(* Logix 5000 AddOnInstructionDefinition export SPEL_Jump; software revision 30.01 *)

ADD_ON_INSTRUCTION SPEL_ExecCmd   (* revision 1.0 *)
// Executes a command in the robot controller.  Normally this is called by higher level AOIs.
VAR_INPUT
   Start : BOOL; {required}
   MaxTime : DINT := 3000; {required}
END_VAR
VAR_OUTPUT
   InCycle : BOOL; {access Read Only, visible}
   Done : BOOL; {access Read Only, visible}
   Error : BOOL; {access Read Only, visible}
END_VAR
VAR_IN_OUT
   ExtInputs : AB:ETHERNET_MODULE_INT_128Bytes:I:0; {required}
        .DATA[0].0   // ExtCmdGet
        .DATA[0].1   // ExtRespSet
        .DATA[0].2   // ExtCmdResult
        .DATA[0].3   // ExtError
   ExtOutputs : AB:ETHERNET_MODULE_INT_128Bytes:O:0; {required}
        .DATA[0].0   // ExtCmdSet
        .DATA[0].1   // ExtRespGet
        .DATA[0].2   // ExtCmdReset
END_VAR
VAR_INPUT
   Cmd : INT; {required}
   CmdParam1 : INT; {required}
   CmdParam2 : INT; {required}
   CmdParam3 : INT; {required}
   CmdParam4 : INT; {required}
   CmdParam5 : INT; {required}
   CmdParam6 : INT; {required}
   CmdParam7 : INT; {required}
END_VAR
VAR_OUTPUT
   CmdEcho : INT; {access Read Only, visible}
   Resp1 : INT; {access Read Only, visible}
   Resp2 : INT; {access Read Only, visible}
   Resp3 : INT; {access Read Only, visible}
   Resp4 : INT; {access Read Only, visible}
   Resp5 : INT; {access Read Only, visible}
   Resp6 : INT; {access Read Only, visible}
   Resp7 : INT; {access Read Only, visible}
   ErrCode1 : INT; {access Read Only, visible}
   ErrCode2 : INT; {access Read Only, visible}
END_VAR
VAR
   ExtReset : BOOL; {access None}
   ExtError : BOOL; {access None}
   ExtCmdSet : BOOL; {access None}   // Cmd Ready
   ExtCmdGet : BOOL; {access None}   // Cmd Received
   CmdXferDone : BOOL; {access None}
   ExtRespSet : BOOL; {access None}   // Resp Ready
   RespXferDone : BOOL; {access None}
   ExtCmdResult : BOOL; {access None}   // Normal or Error?
   TmrCmdDataRdy : TIMER := (PRE := 5); {access None}
   OneShotDoneOff : BOOL; {access None}
   OneShotStart : BOOL; {access None}
   StartInit : BOOL; {access None}
   OneShotStartError : BOOL; {access None}
   TmrCycle : TIMER := (PRE := 5000); {access None}
   OneshotTmrPreset : BOOL; {access None}
   TmrCmdSet : TIMER := (PRE := 20); {access None}
   OnShotCmdDataXfer : BOOL; {access None}
   OneShotRespDataXfer : BOOL; {access None}
   OneShotDataRdy : BOOL; {access None}
   OtherCmdInCycle : BOOL; {access None}
   s : BOOL; {access None}
   OneShotUnsetCmdIncycle : BOOL; {access None}
   OneShotSetCmdIncycle : BOOL; {access None}
   OneShotSetOtherCmdInCycleError : BOOL; {access None}
   OneShotSetBit : BOOL; {access None}
   MaxTimeError : BOOL; {access None}
END_VAR

ROUTINE Logic   (* ladder *)
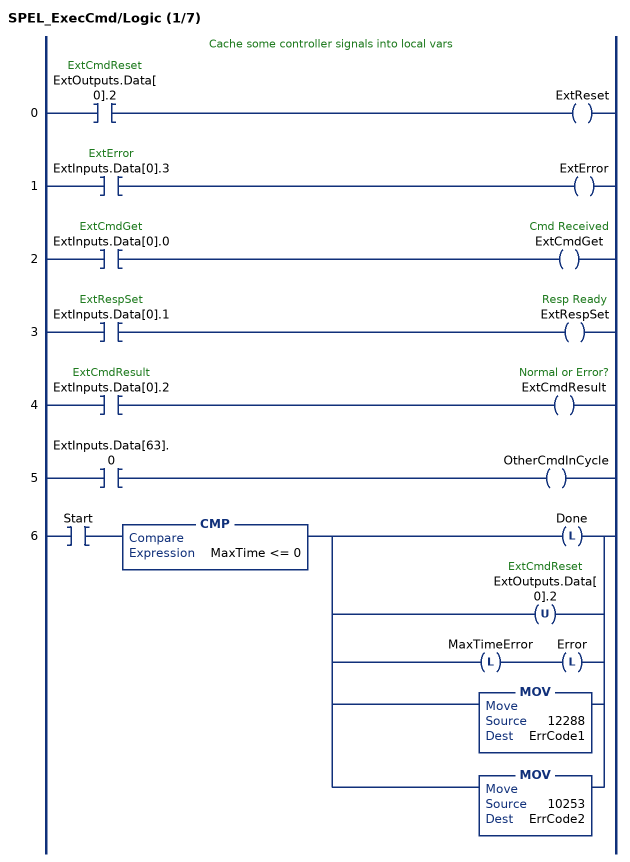
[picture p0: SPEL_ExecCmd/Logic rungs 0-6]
   // Cache some controller signals into local vars
   0: XIC(ExtOutputs.Data[0].2)OTE(ExtReset);
   1: XIC(ExtInputs.Data[0].3)OTE(ExtError);
   2: XIC(ExtInputs.Data[0].0)OTE(ExtCmdGet);
   3: XIC(ExtInputs.Data[0].1)OTE(ExtRespSet);
   4: XIC(ExtInputs.Data[0].2)OTE(ExtCmdResult);
   5: XIC(ExtInputs.Data[63].0)OTE(OtherCmdInCycle);
   6: XIC(Start)CMP(MaxTime <= 0)[OTL(Done) ,OTU(ExtOutputs.Data[0].2) ,OTL(MaxTimeError) OTL(Error) ,MOV(12288,ErrCode1) ,MOV(10253,ErrCode2) ];
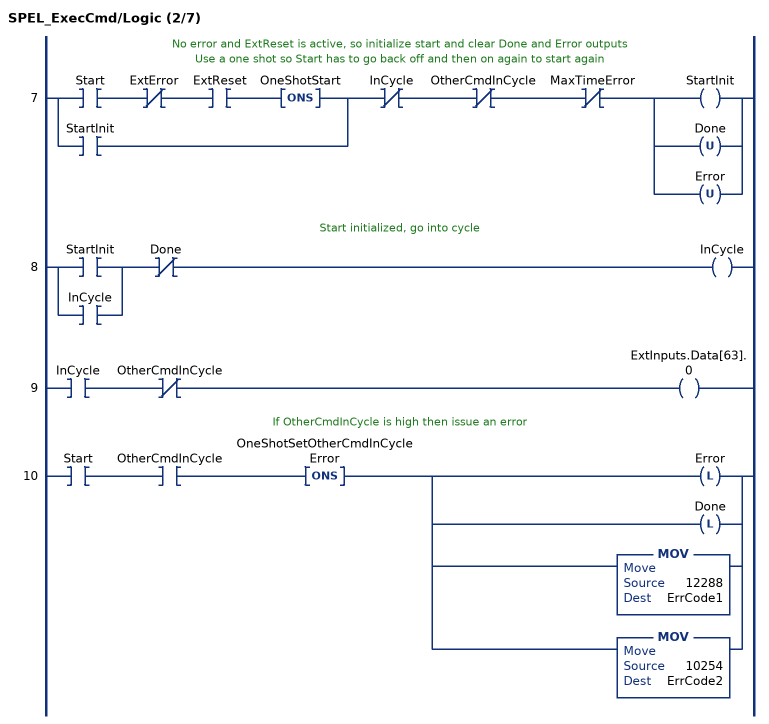
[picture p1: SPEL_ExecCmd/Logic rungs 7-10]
   // No error and ExtReset is active, so initialize start and clear Done and Error outputs
   // Use a one shot so Start has to go back off and then on again to start again
   7: [XIC(Start) XIO(ExtError) XIC(ExtReset) ONS(OneShotStart) ,XIC(StartInit) ]XIO(InCycle)XIO(OtherCmdInCycle)XIO(MaxTimeError)[OTE(StartInit) ,OTU(Done) ,OTU(Error) ];
   // Start initialized, go into cycle
   8: [XIC(StartInit) ,XIC(InCycle) ]XIO(Done)OTE(InCycle);
   9: XIC(InCycle)XIO(OtherCmdInCycle)OTE(ExtInputs.Data[63].0);
   // If OtherCmdInCycle is high then issue an error
   10: XIC(Start)XIC(OtherCmdInCycle)ONS(OneShotSetOtherCmdInCycleError)[OTL(Error) ,OTL(Done) ,MOV(12288,ErrCode1) ,MOV(10254,ErrCode2) ];
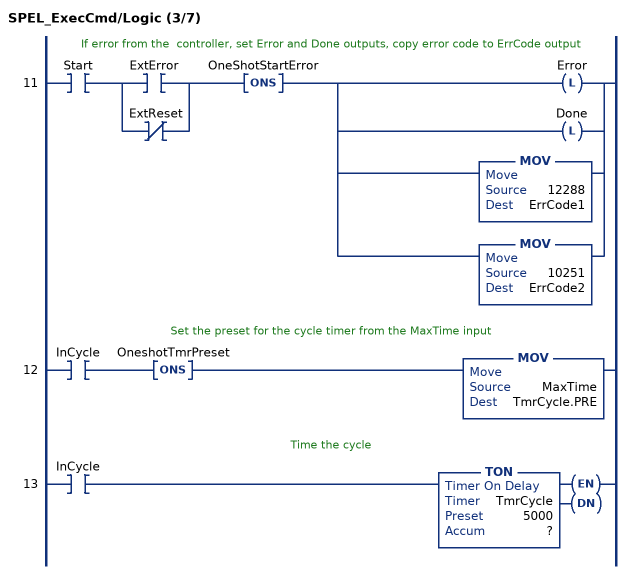
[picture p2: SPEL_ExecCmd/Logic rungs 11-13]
   // If error from the  controller, set Error and Done outputs, copy error code to ErrCode output
   11: XIC(Start)[XIC(ExtError) ,XIO(ExtReset) ]ONS(OneShotStartError)[OTL(Error) ,OTL(Done) ,MOV(12288,ErrCode1) ,MOV(10251,ErrCode2) ];
   // Set the preset for the cycle timer from the MaxTime input
   12: XIC(InCycle)ONS(OneshotTmrPreset)MOV(MaxTime,TmrCycle.PRE);
   // Time the cycle
   13: XIC(InCycle)TON(TmrCycle,?,?);
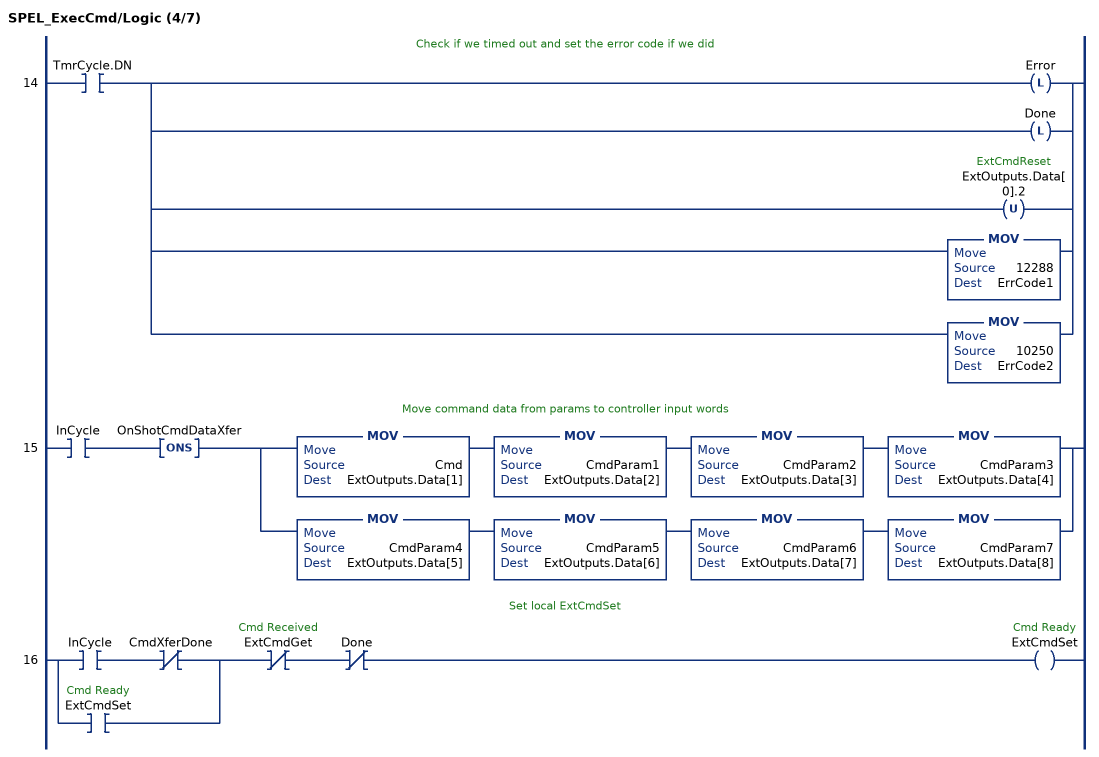
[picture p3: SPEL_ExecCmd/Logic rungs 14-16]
   // Check if we timed out and set the error code if we did
   14: XIC(TmrCycle.DN)[OTL(Error) ,OTL(Done) ,OTU(ExtOutputs.Data[0].2) ,MOV(12288,ErrCode1) ,MOV(10250,ErrCode2) ];
   // Move command data from params to controller input words
   15: XIC(InCycle)ONS(OnShotCmdDataXfer)[MOV(Cmd,ExtOutputs.Data[1]) MOV(CmdParam1,ExtOutputs.Data[2]) MOV(CmdParam2,ExtOutputs.Data[3]) MOV(CmdParam3,ExtOutputs.Data[4]) ,MOV(CmdParam4,ExtOutputs.Data[5]) MOV(CmdParam5,ExtOutputs.Data[6]) MOV(CmdParam6,ExtOutputs.Data[7]) MOV(CmdParam7,ExtOutputs.Data[8]) ];
   // Set local ExtCmdSet
   16: [XIC(InCycle) XIO(CmdXferDone) ,XIC(ExtCmdSet) ]XIO(ExtCmdGet)XIO(Done)OTE(ExtCmdSet);
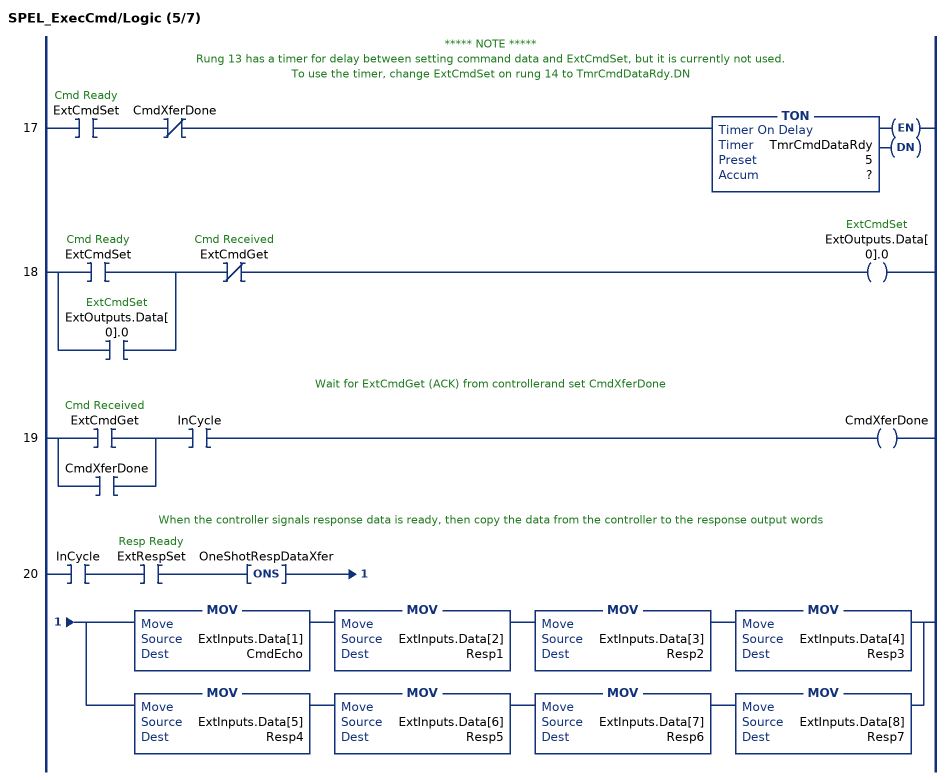
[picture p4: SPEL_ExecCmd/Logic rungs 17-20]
   // ***** NOTE *****
   // Rung 13 has a timer for delay between setting command data and ExtCmdSet, but it is currently not used.
   // To use the timer, change ExtCmdSet on rung 14 to TmrCmdDataRdy.DN
   17: XIC(ExtCmdSet)XIO(CmdXferDone)TON(TmrCmdDataRdy,?,?);
   18: [XIC(ExtCmdSet) ,XIC(ExtOutputs.Data[0].0) ]XIO(ExtCmdGet)OTE(ExtOutputs.Data[0].0);
   // Wait for ExtCmdGet (ACK) from controllerand set CmdXferDone
   19: [XIC(ExtCmdGet) ,XIC(CmdXferDone) ]XIC(InCycle)OTE(CmdXferDone);
   // When the controller signals response data is ready, then copy the data from the controller to the response output words
   20: XIC(InCycle)XIC(ExtRespSet)ONS(OneShotRespDataXfer)[MOV(ExtInputs.Data[1],CmdEcho) MOV(ExtInputs.Data[2],Resp1) MOV(ExtInputs.Data[3],Resp2) MOV(ExtInputs.Data[4],Resp3) ,MOV(ExtInputs.Data[5],Resp4) MOV(ExtInputs.Data[6],Resp5) MOV(ExtInputs.Data[7],Resp6) MOV(ExtInputs.Data[8],Resp7) ];
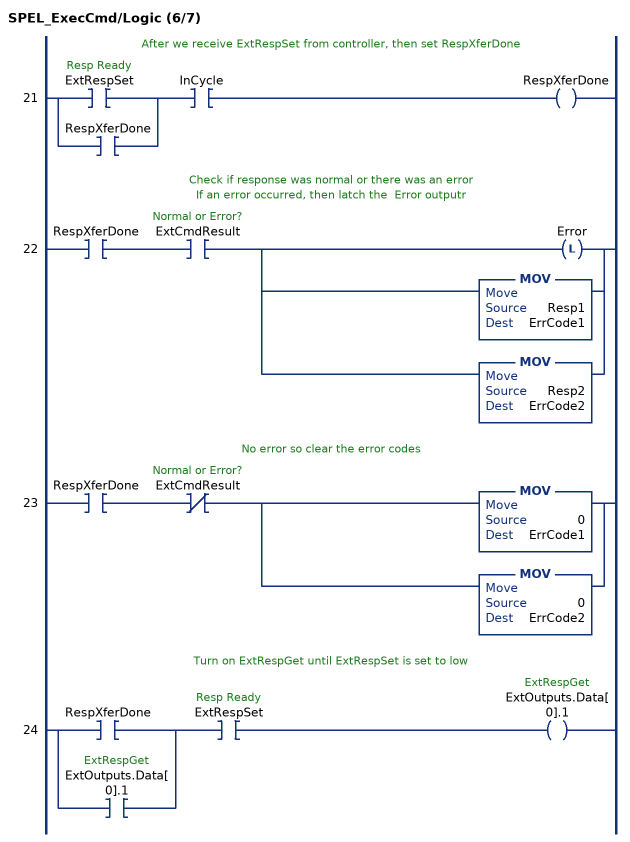
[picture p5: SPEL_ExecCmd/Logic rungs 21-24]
   // After we receive ExtRespSet from controller, then set RespXferDone
   21: [XIC(ExtRespSet) ,XIC(RespXferDone) ]XIC(InCycle)OTE(RespXferDone);
   // Check if response was normal or there was an error
   // If an error occurred, then latch the  Error outputr
   22: XIC(RespXferDone)XIC(ExtCmdResult)[OTL(Error) ,MOV(Resp1,ErrCode1) ,MOV(Resp2,ErrCode2) ];
   // No error so clear the error codes
   23: XIC(RespXferDone)XIO(ExtCmdResult)[MOV(0,ErrCode1) ,MOV(0,ErrCode2) ];
   // Turn on ExtRespGet until ExtRespSet is set to low
   24: [XIC(RespXferDone) ,XIC(ExtOutputs.Data[0].1) ]XIC(ExtRespSet)OTE(ExtOutputs.Data[0].1);
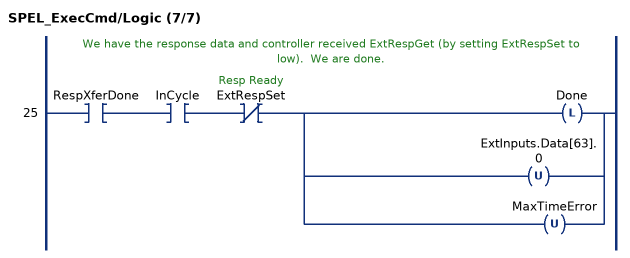
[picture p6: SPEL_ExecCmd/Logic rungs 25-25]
   // We have the response data and controller received ExtRespGet (by setting ExtRespSet to low).  We are done.
   25: XIC(RespXferDone)XIC(InCycle)XIO(ExtRespSet)[OTL(Done) ,OTU(ExtInputs.Data[63].0) ,OTU(MaxTimeError) ];
END_ROUTINE
END_ADD_ON_INSTRUCTION

ADD_ON_INSTRUCTION SPEL_Jump   (* revision 1.0, vendor SEIKO EPSON CORP. *)
// Moves the arm in gate trajectory using PTP motion.
VAR_OUTPUT
   InCycle : BOOL; {access Read Only, visible}
   Done : BOOL; {access Read Only, visible}
   Error : BOOL; {access Read Only, visible}
END_VAR
VAR_INPUT
   Start : BOOL; {required}
   MaxTime : DINT := 30000; {access None, visible}
   TargetType : INT; {access None, visible}
   ArchNum : INT := 7; {access None, visible}
   Point : INT; {required}
   PalletNum : INT; {access None, visible}
   PalletPosOrCol : INT; {access None, visible}
   PalletRow : INT; {access None, visible}
END_VAR
VAR_IN_OUT
   ExtInputs : AB:ETHERNET_MODULE_INT_128Bytes:I:0; {required}
   ExtOutputs : AB:ETHERNET_MODULE_INT_128Bytes:O:0; {required}
END_VAR
VAR_OUTPUT
   ErrCode1 : INT; {access Read Only, visible}
   ErrCode2 : INT; {access Read Only, visible}
END_VAR
VAR
   ExecJump : SPEL_ExecCmd := (MaxTime := 3000, CmdParam1 := 112); {access None}
   StartInit : BOOL; {access None}
   CmdParam1 : INT; {access None}
   PointOrPalletNum : INT; {access None}
   BSL_Control : CONTROL; {access None}
   BSL_SourceBit : BOOL; {access None}
   Local_Arch : DINT; {access None}
   OneShotStart : BOOL; {access None}
   ExecTimeout : DINT; {access None}
   OneShotCP : BOOL; {access None}
   Local_CP : DINT; {access None}
   LocalCP : DINT; {access None}
   ArchError : BOOL; {access None}
   StartExec : BOOL; {access None}
   ExecuteCmd : BOOL; {access None}
   TargetTypeError : BOOL; {access None}
   OneShotArch : BOOL; {access None}
   OneShotTargetType : BOOL; {access None}
END_VAR

ROUTINE Logic   (* ladder *)
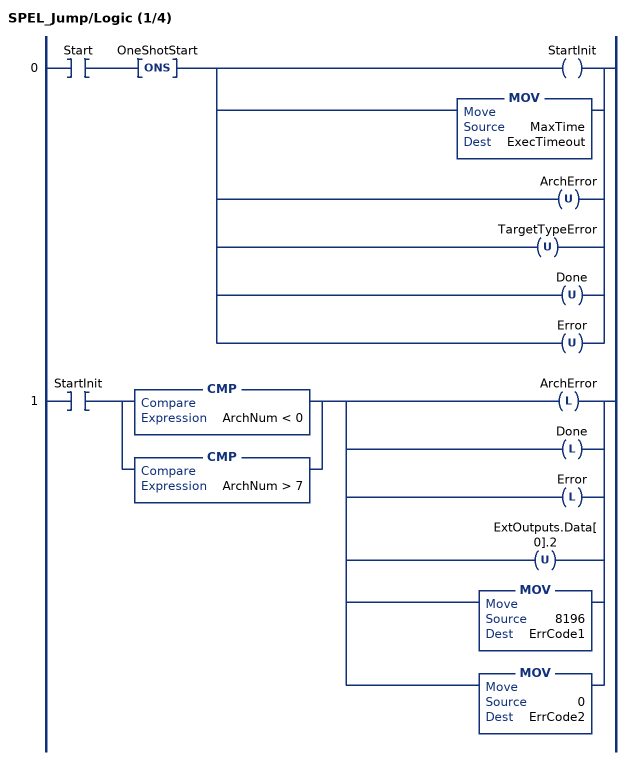
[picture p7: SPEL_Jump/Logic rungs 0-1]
   0: XIC(Start)ONS(OneShotStart)[OTE(StartInit) ,MOV(MaxTime,ExecTimeout) ,OTU(ArchError) ,OTU(TargetTypeError) ,OTU(Done) ,OTU(Error) ];
   1: XIC(StartInit)[CMP(ArchNum < 0) ,CMP(ArchNum > 7) ][OTL(ArchError) ,OTL(Done) ,OTL(Error) ,OTU(ExtOutputs.Data[0].2) ,MOV(8196,ErrCode1) ,MOV(0,ErrCode2) ];
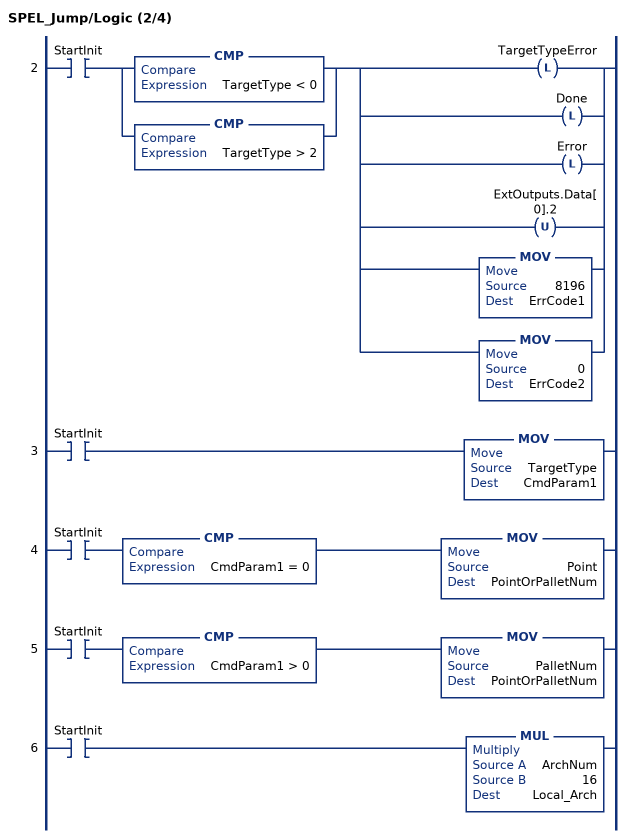
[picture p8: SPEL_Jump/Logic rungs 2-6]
   2: XIC(StartInit)[CMP(TargetType < 0) ,CMP(TargetType > 2) ][OTL(TargetTypeError) ,OTL(Done) ,OTL(Error) ,OTU(ExtOutputs.Data[0].2) ,MOV(8196,ErrCode1) ,MOV(0,ErrCode2) ];
   3: XIC(StartInit)MOV(TargetType,CmdParam1);
   4: XIC(StartInit)CMP(CmdParam1 = 0)MOV(Point,PointOrPalletNum);
   5: XIC(StartInit)CMP(CmdParam1 > 0)MOV(PalletNum,PointOrPalletNum);
   6: XIC(StartInit)MUL(ArchNum,16,Local_Arch);
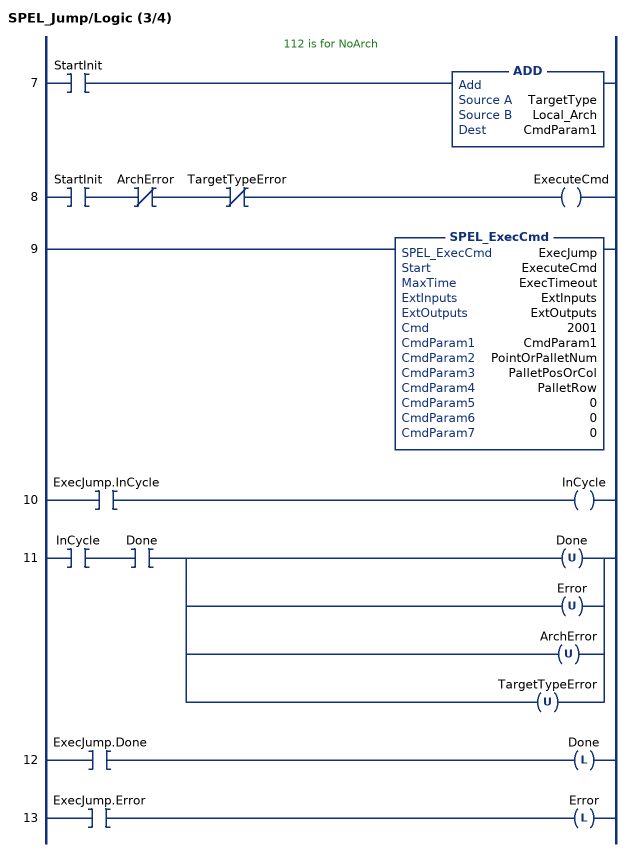
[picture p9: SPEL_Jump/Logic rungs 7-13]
   // 112 is for NoArch
   7: XIC(StartInit)ADD(TargetType,Local_Arch,CmdParam1);
   8: XIC(StartInit)XIO(ArchError)XIO(TargetTypeError)OTE(ExecuteCmd);
   9: SPEL_ExecCmd(ExecJump,ExecuteCmd,ExecTimeout,ExtInputs,ExtOutputs,2001,CmdParam1,PointOrPalletNum,PalletPosOrCol,PalletRow,0,0,0);
   10: XIC(ExecJump.InCycle)OTE(InCycle);
   11: XIC(InCycle)XIC(Done)[OTU(Done) ,OTU(Error) ,OTU(ArchError) ,OTU(TargetTypeError) ];
   12: XIC(ExecJump.Done)OTL(Done);
   13: XIC(ExecJump.Error)OTL(Error);
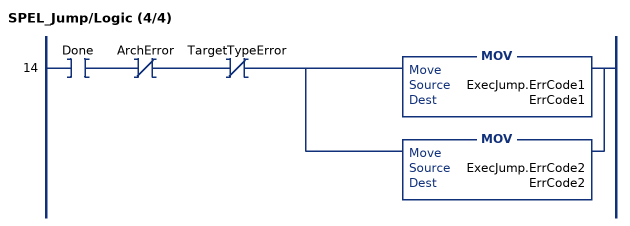
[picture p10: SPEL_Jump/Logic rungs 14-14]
   14: XIC(Done)XIO(ArchError)XIO(TargetTypeError)[MOV(ExecJump.ErrCode1,ErrCode1) ,MOV(ExecJump.ErrCode2,ErrCode2) ];
END_ROUTINE
END_ADD_ON_INSTRUCTION
